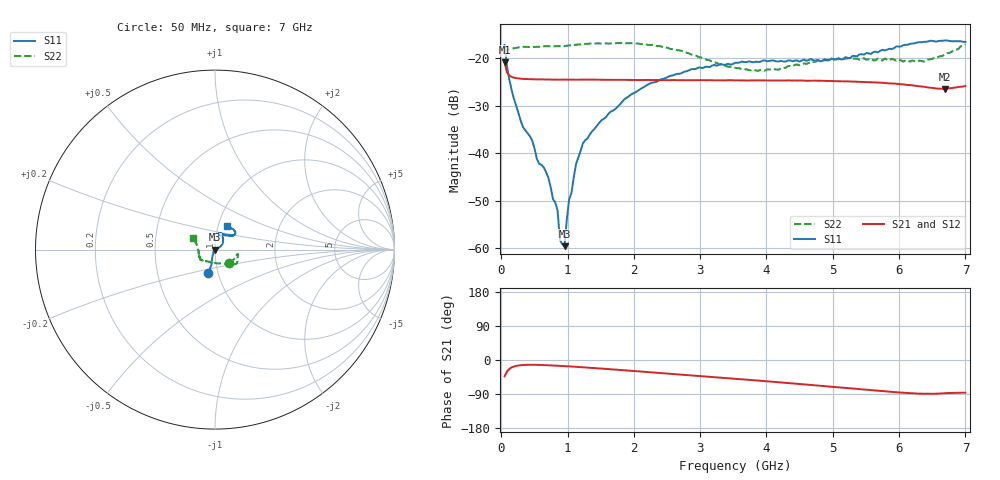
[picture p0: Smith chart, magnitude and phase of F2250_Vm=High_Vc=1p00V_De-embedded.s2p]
! Integrated Device Technology
! Corporate Headquarters
! 6024 Silver Creek Valley Road
! San Jose, CA 95138  USA
! Phone:  1-408-284-8200
! Toll Free:  1-800-223-1366
! Webpage:  http://www.idt.com/
! Timing and RF Division
! 515 Groton Road, Suite 102
! Westford, MA 01886-6024
! Device:  F2250
! Description: Voltage Variable RF Attenuator
! Frequency:  50.0 -  6000.00 MHz
! Package:  3x3 mm Thin QFN Plastic Package: 16 pin
! Ports:  2 RF, 3 DC
!  Pin  1  = GND
!  Pin  2  = NC
!  Pin  3  = RF1  = Port 1
!  Pin  4  = NC
!  Pin  5  = GND
!  Pin  6  = GND
!  Pin  7  = GND
!  Pin  8  = GND
!  Pin  9  = NC
!  Pin 10  = RF2  = Port 2
!  Pin 11  = NC
!  Pin 12  = GND
!  Pin 13  = GND
!  Pin 14  = VCNTRL
!  Pin 15  = VDD
!  Pin 16  = VMODE
! Vcntrl:  1.000 Volts
! Vmode:  +3.300 Volts
! Vdd:  +3.30  Volts
! Current:  1.325 mA
! Data:  The device was measured on a the F2250 evaluation board which has
!  individual transmission lines to the RF pins.  Data was collected
!  using a calibrated network analyzer.  The evaluation board was
!  de-embedded using a TRL calibration technique.
!  The reference plane is the edge of the package pin.
! Misc:  SN 10
!  Action Tracker AT0258
! Date Measured:  2014-11-26
! Date:  2015-10-15  MJV
! Note:
!  Integrated Device Technology supplies this data as a sample of measured
!  data at the package pin for this product.  Your particular data for this
!  product may vary.
!  Data was taken at 25 degrees C.
!  Integrated Device Technology reserves the right to change this data at anytime.
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# GHz S dB R 50
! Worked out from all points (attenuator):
!   201 points, 50 MHz to 7 GHz, reference 50 ohm
!   highest |S21| = -20.94 dB at 50 MHz (marker M1); lowest = -26.5 dB at 6.687 GHz (marker M2)
!   lowest |S11| = -59.5 dB at 953.5 MHz (marker M3), VSWR 1.00, Z = 49.9 - j0.091 ohm
!   |S11| at or under -10 dB: start of sweep to end of sweep
!   |S22| runs from -22.7 to -16.9 dB; largest |S21 - S12| = 0.00029
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0.05  -17.26 -105.6  -20.94 -42.9  -20.95 -42.9  -19.11 -43.3
0.1195  -24.45 -106.5  -23.66 -23.7  -23.66 -23.7  -18.16 -15.7
0.189  -28.51 -111.7  -24.14 -17.2  -24.14 -17.2  -17.97 -12.1
0.328  -34.53 -119.5  -24.40 -13.2  -24.39 -13.2  -17.67 -11.0
0.467  -37.35 -128.6  -24.48 -12.6  -24.46 -12.7  -17.73 -12.2
0.5365  -41.19 -131.2  -24.49 -12.8  -24.48 -12.8  -17.66 -13.7
0.71025  -45.18 -139.6  -24.54 -13.9  -24.54 -13.9  -17.54 -16.7
0.84925  -52.05 -174.3  -24.57 -15.1  -24.56 -15.1  -17.52 -19.7
0.884  -58.21 179.4  -24.58 -15.5  -24.56 -15.5  -17.48 -20.6
0.9535  -59.52 -120.5  -24.56 -16.1  -24.56 -16.1  -17.51 -21.5
1.023  -49.75 -2.6  -24.57 -16.8  -24.55 -16.8  -17.37 -22.3
1.05775  -48.35 6.4  -24.56 -17.2  -24.56 -17.2  -17.35 -22.5
1.12725  -42.29 12.5  -24.57 -18.0  -24.57 -18.0  -17.23 -24.0
1.2315  -37.92 16.2  -24.56 -19.2  -24.55 -19.2  -17.05 -26.0
1.857  -28.68 30.7  -24.60 -27.1  -24.60 -27.2  -16.88 -32.7
2.37825  -24.72 41.1  -24.67 -33.9  -24.66 -33.9  -17.47 -37.8
3.525  -21.03 69.1  -24.71 -49.5  -24.70 -49.6  -22.08 -77.8
4.18525  -20.73 75.8  -24.77 -58.6  -24.75 -58.7  -22.47 -119.1
4.7065  -20.52 70.6  -24.79 -66.5  -24.79 -66.5  -20.85 -137.7
5.85325  -18.07 39.2  -25.35 -83.6  -25.33 -83.7  -20.55 -157.4
6.68725  -16.34 47.0  -26.51 -87.7  -26.48 -87.9  -19.30 162.4
7  -16.64 61.9  -25.89 -86.2  -25.88 -86.4  -17.15 153.5
